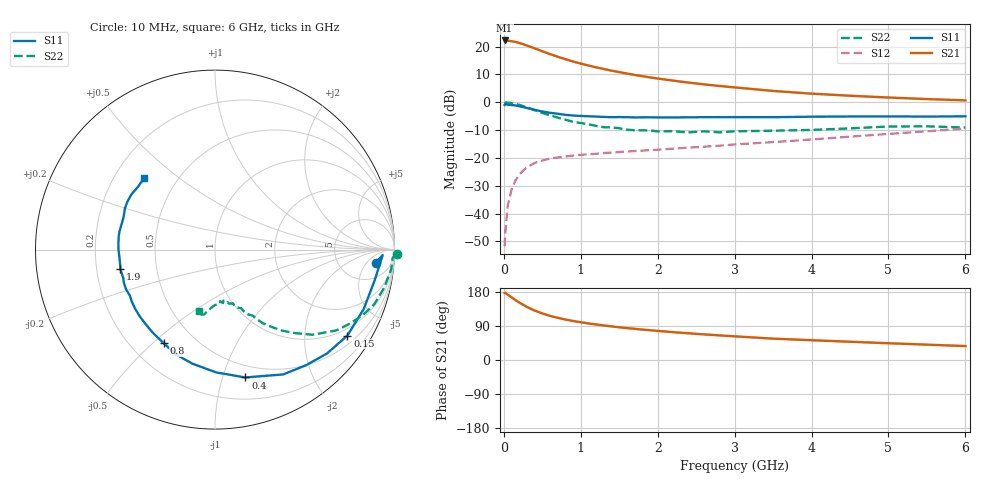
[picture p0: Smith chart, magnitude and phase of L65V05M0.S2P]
!  INFINEON TECHNOLOGIES Small Signal Semiconductors
! BFR380L3 , Si-NPN RF-Transistor in TSLP-3-1
!  Vce=5 V,  Ic=5 mA
! Common Emitter S-Parameters:  07. March 2005
#  GHz  S  MA  R  50
! f  S11  S21  S12  S22
! GHz  Mag  Ang  Mag  Ang  Mag  Ang  Mag  Ang
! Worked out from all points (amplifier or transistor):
!   36 points, 10 MHz to 6 GHz, reference 50 ohm
!   highest |S21| = 22.2 dB at 10 MHz (marker M1)
!   |S21| within 3 dB of that: start of sweep to 416.8 MHz
!   unconditionally stable (mu >= 1): 2.701 GHz to 4.579 GHz
!   at 250 MHz: K = 0.15, MSG = 22.7 dB, |S12| = -24.5 dB
!   at 1.4 GHz: K = 0.72, MSG = 14.7 dB, |S12| = -18.1 dB
!   at 6 GHz: K = 0.92, MSG = 5.1 dB, |S12| = -9.4 dB
!   S11 on the Smith chart (normalised r, x): 10 MHz: 12, -9; 150 MHz: 0.76, -3.21; 400 MHz: 0.39, -1.19; 800 MHz: 0.34, -0.54; 1.9 GHz: 0.30, -0.09; 6 GHz: 0.33, +0.38
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0.01  0.8981 -4.6  12.92 176.7  0.0026 78.8  1.012 -1.3
0.02  0.9349 -1.9  12.88 177.2  0.0047 90.0  0.9907 -2.7
0.05  0.9051 -11.2  12.8 172.5  0.0137 86.9  0.9877 -6.5
0.1  0.8922 -21.8  12.51 165.4  0.027 78.9  0.9656 -12.8
0.15  0.8795 -33.0  12.17 158.3  0.0393 72.6  0.9379 -19.0
0.2  0.8509 -42.9  11.66 151.6  0.0503 69.3  0.9002 -24.0
0.25  0.8199 -51.8  11.09 145.9  0.0593 63.9  0.8529 -29.2
0.3  0.7926 -61.3  10.48 140.0  0.0678 60.2  0.8117 -33.7
0.4  0.7324 -76.6  9.336 130.5  0.0812 53.9  0.7216 -41.1
0.5  0.6844 -89.4  8.274 123.0  0.0899 49.6  0.6459 -46.1
0.6  0.6479 -101.2  7.347 116.4  0.0971 46.3  0.5844 -50.5
0.8  0.5949 -118.7  5.957 106.8  0.1063 42.8  0.4861 -57.2
0.9  0.5786 -126.7  5.411 102.9  0.1103 41.9  0.4464 -59.2
1.1  0.5611 -138.0  4.579 96.4  0.1167 41.7  0.4028 -63.2
1.5  0.5429 -155.9  3.49 86.3  0.1277 42.9  0.3427 -69.4
1.9  0.538 -168.5  2.801 78.5  0.1381 45.0  0.3114 -75.4
2.2  0.5343 -175.7  2.454 73.5  0.147 47.2  0.3025 -77.1
2.8  0.5416 171.8  1.968 65.0  0.166 51.6  0.2888 -84.3
3.5  0.5401 160.8  1.6 56.4  0.1925 54.9  0.3087 -89.9
4.5  0.5562 151.6  1.312 48.2  0.2413 59.6  0.3398 -96.1
5.5  0.5539 141.1  1.143 40.5  0.3017 60.6  0.3699 -101.9
6  0.5603 134.8  1.083 36.8  0.3376 59.9  0.3526 -104.4
